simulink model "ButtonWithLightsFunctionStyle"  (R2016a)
settings: Solver=FixedStepAuto  StartTime=0.0  StopTime=inf  RelTol=1e-3
libraries: miniQ x2

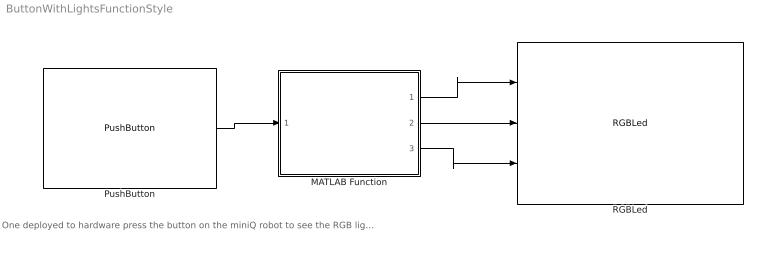
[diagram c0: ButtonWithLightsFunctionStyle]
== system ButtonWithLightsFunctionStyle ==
  note: One deployed to hardware press the button on the miniQ robot to see the RGB light turn on. The color of the light can be changed by clicking into the MATLAB function block then changing some of the variables.
  MATLAB Function : MATLAB Function  TreatAsAtomicUnit=on
  PushButton : miniQ/PushButton  sampleTime_dd=0.1  debug_dd=off
  RGBLed : miniQ/RGBLed
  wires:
  PushButton/1 -> MATLAB Function/1(button)
  MATLAB Function/2(green) -> RGBLed/2
  MATLAB Function/3(blue) -> RGBLed/3
  MATLAB Function/1(red) -> RGBLed/1

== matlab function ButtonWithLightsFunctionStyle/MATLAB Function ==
function [red,green,blue] = fcn(button)
if button==1 %each button outputs it's value. >0 means that any of the three buttons on the miniQ can be pressed
    red=200;
    green=0;
    blue=0;
elseif button == 2
    red=0;
    green=0;
    blue=200;
elseif button ==3
    red=0;
    green=255;
    blue =0;
else
    red=0;
    green=0;
    blue =0;
end
end
